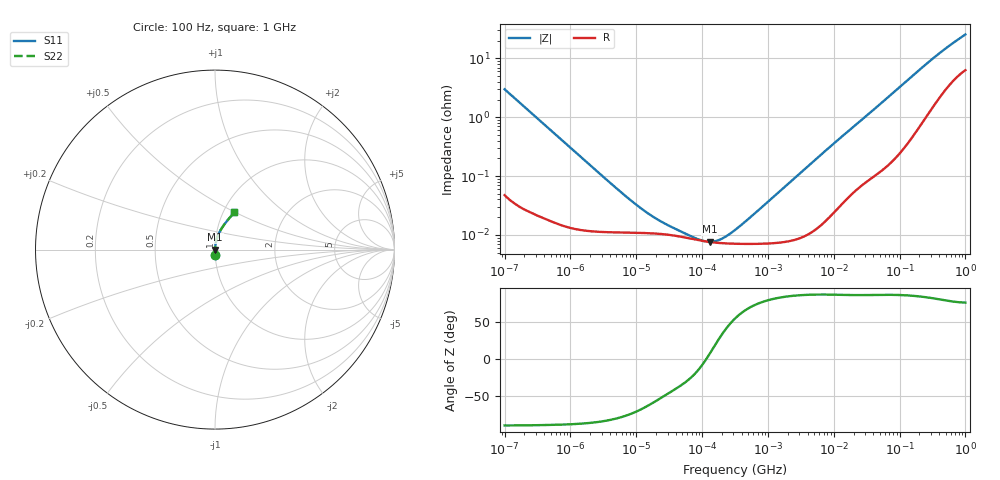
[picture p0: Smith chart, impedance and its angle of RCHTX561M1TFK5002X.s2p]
! RCHTX561M1TFK5002X  S-PARAMETER MODEL  (AEC-Q200 qualified)
! Model Generated by ELNA Corporation (http://www.ty-top.com)
! Version 1.0
! ELNA Control No. 231122
! Copyright (c) 2023 ELNA CO.,LTD. All Rights Reserved.
! Products Name : CONDUCTIVE POLYMER HYBRID ALUMINUM ELECTROLYTIC CAPACITORS
! Characteristics :
!  Capacitance  :  560uF  ,  Rated voltage  :  25V
!  Operating Temp. Range  :  -55 to +135 degC  ,  Endurance  :  4000hr at 135 degC
!  Dimension D  :  10mm  ,  Dimension L  :  12.5mm
! Frequency Range : 100Hz - 1GHz
! External Node Assignments :
!  1  o---| |---o  2
# MHz S RI R 50
!Freq[MHz].  S11 Real  S11 Imag  S21 Real  S21 Imag  S12 Real  S12 Imag  S22 Real  S22 Imag
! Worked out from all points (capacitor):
!   401 points, 100 Hz to 1 GHz, reference 50 ohm
!   read as one part in series: C = 532 uF near 108 Hz
!   lowest |Z| = 7.63 mohm at 130.3 kHz (marker M1)
!   series resonance near 116.1 kHz, so ESL is about 3.5 nH
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0.0001  0.00136 -0.0298  0.9986 0.0298  0.9986 0.0298  0.00136 -0.0298
0.000113  0.00112 -0.0265  0.9989 0.0265  0.9989 0.0265  0.00112 -0.0265
0.000309  0.000309 -0.00971  0.9997 0.00971  0.9997 0.00971  0.000309 -0.00971
0.001488  0.000124 -0.00204  0.9999 0.00204  0.9999 0.00204  0.000124 -0.00204
0.004241  0.000111 -0.000718  0.9999 0.000718  0.9999 0.000718  0.000111 -0.000718
0.008414  0.000109 -0.000364  0.9999 0.000364  0.9999 0.000364  0.000109 -0.000364
0.014207  0.000107 -0.000218  0.9999 0.000218  0.9999 0.000218  0.000107 -0.000218
0.022131  0.000104 -0.000143  0.9999 0.000143  0.9999 0.000143  0.000104 -0.000143
0.034475  9.88e-05 -9.34e-05  0.9999 9.34e-05  0.9999 9.34e-05  9.88e-05 -9.34e-05
0.060604  8.82e-05 -4.82e-05  0.9999 4.82e-05  0.9999 4.82e-05  8.82e-05 -4.82e-05
0.130317  7.57e-05 9.16e-06  0.9999 -9.16e-06  0.9999 -9.16e-06  7.57e-05 9.16e-06
0.238506  7.15e-05 6.47e-05  0.9999 -6.47e-05  0.9999 -6.47e-05  7.15e-05 6.47e-05
0.269153  7.11e-05 7.82e-05  0.9999 -7.82e-05  0.9999 -7.82e-05  7.11e-05 7.82e-05
0.316228  7.07e-05 9.81e-05  0.9999 -9.81e-05  0.9999 -9.81e-05  7.07e-05 9.81e-05
0.653131  7.04e-05 0.000229  0.9999 -0.000229  0.9999 -0.000229  7.04e-05 0.000229
4.704354  0.000115 0.0017  0.9999 -0.0017  0.9999 -0.0017  0.000115 0.0017
69.9842  0.00211 0.0227  0.9979 -0.0227  0.9979 -0.0227  0.00211 0.0227
163.1173  0.00755 0.0515  0.9925 -0.0515  0.9925 -0.0515  0.00755 0.0515
350.7519  0.0276 0.1019  0.9724 -0.1019  0.9724 -0.1019  0.0276 0.1019
616.595  0.0626 0.1542  0.9374 -0.1542  0.9374 -0.1542  0.0626 0.1542
922.5714  0.0992 0.1978  0.9008 -0.1978  0.9008 -0.1978  0.0992 0.1978
1000  0.1075 0.2074  0.8925 -0.2074  0.8925 -0.2074  0.1075 0.2074
